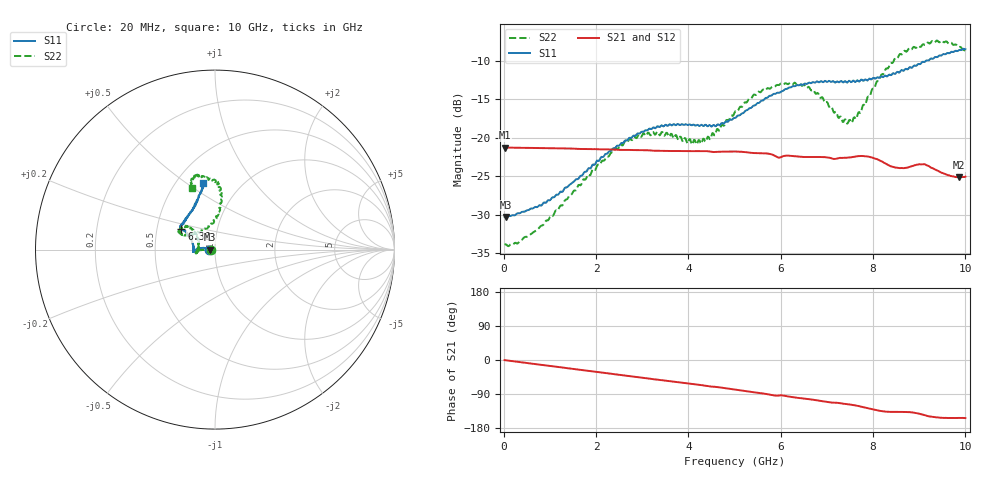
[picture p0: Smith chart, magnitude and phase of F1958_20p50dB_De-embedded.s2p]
! Integrated Device Technology
! Corporate Headquarters
! 6024 Silver Creek Valley Road
! San Jose, CA 95138  USA
! Phone:  1-408-284-8200
! Toll Free:  1-800-223-1366
! Webpage:  http://www.idt.com/
! Timing and RF Division
! 515 Groton Road, Suite 102
! Westford, MA 01886-6024
! Device:  F1958
! Description: 7-bit 0.25 dB Digital Step Attenuator
! Frequency:  0.001 -  6.000 GHz
! Package:  4x4 mm Thin QFN Plastic Package: 24 pin
! Ports:  2 RF, 12 DC
!  Pin  1  = D0
!  Pin  2  = VDD
!  Pin  3  = VMODE
!  Pin  4  = GND
!  Pin  5  = RF1  =  Port 1
!  Pin  6  = GND
!  Pin  7  = GND
!  Pin  8  = GND
!  Pin  9  = GND
!  Pin 10  = GND
!  Pin 11  = GND
!  Pin 12  = GND
!  Pin 13  = GND
!  Pin 14  = RF2  =  Port 2
!  Pin 15  = GND
!  Pin 16  = LE
!  Pin 17  = CLK
!  Pin 18  = DATA
!  Pin 19  = D6
!  Pin 20  = D5
!  Pin 21  = D4
!  Pin 22  = D3
!  Pin 23  = D2
!  Pin 24  = D1
! State:  82
! Atten State:  20.50 dB
! Voltage:  +3.30 Volts
! Current:  0.258 mA
! Data:  The device was measured on a F1958 evaluation board which has
!  individual transmission lines to the RF pins.  Data was collected
!  using a calibrated network analyzer.  The evaluation board was
!  de-embedded using Automatic Fixture Removal (AFR).
!  The reference plane is the edge of the package pin.
! Misc:
!  Action Tracker AT0419
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# GHz S dB R 50
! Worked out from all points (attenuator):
!   500 points, 20 MHz to 10 GHz, reference 50 ohm
!   highest |S21| = -21.27 dB at 20 MHz (marker M1); lowest = -25.1 dB at 9.86 GHz (marker M2)
!   lowest |S11| = -30.3 dB at 40 MHz (marker M3), VSWR 1.06, Z = 47 - j0.042 ohm
!   |S11| at or under -10 dB: start of sweep to 9.144 GHz
!   |S22| runs from -34.1 to -7.3 dB; largest |S21 - S12| = 0.00033
!   S11 on the Smith chart (normalised r, x): 20 MHz: 0.94, -0.00; 6.36 GHz: 0.67, +0.16; 10 GHz: 0.68, +0.58
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0.02  -30.27 -178.9  -21.27 -0.4  -21.27 -0.4  -33.91 -178.0
0.04  -30.30 -179.2  -21.27 -0.7  -21.27 -0.7  -33.85 -177.0
0.32  -29.82 175.3  -21.31 -5.1  -21.30 -5.1  -33.64 178.7
0.72  -29.03 172.9  -21.33 -11.4  -21.33 -11.4  -31.97 180.0
1.7  -24.90 171.4  -21.45 -26.5  -21.45 -26.5  -25.75 179.3
2.6  -20.60 177.3  -21.58 -40.4  -21.56 -40.4  -20.76 -176.4
3.36  -18.59 -175.3  -21.70 -52.3  -21.70 -52.4  -19.52 -168.5
4.24  -18.48 -178.7  -21.74 -65.7  -21.75 -65.7  -20.32 169.3
4.52  -18.48 174.4  -21.86 -70.2  -21.87 -70.3  -19.39 153.9
5.02  -17.41 161.1  -21.79 -78.0  -21.81 -78.0  -16.53 139.4
5.58  -15.17 150.8  -22.01 -87.5  -22.03 -87.6  -13.99 139.6
6.36  -13.15 148.2  -22.44 -99.8  -22.46 -99.7  -13.15 153.1
6.68  -12.81 146.7  -22.49 -104.5  -22.51 -104.4  -13.81 154.3
7.3  -12.61 140.9  -22.62 -114.3  -22.62 -114.1  -17.24 134.0
7.5  -12.64 138.3  -22.57 -117.5  -22.56 -117.4  -17.67 115.5
7.68  -12.60 135.4  -22.39 -121.4  -22.39 -121.3  -16.71 98.0
8.34  -11.81 119.2  -23.58 -136.8  -23.58 -136.9  -10.81 82.6
8.68  -11.18 112.5  -23.94 -137.3  -23.95 -137.1  -8.68 87.1
9.06  -10.16 106.9  -23.46 -143.7  -23.47 -143.7  -7.97 95.2
9.26  -9.69 104.8  -23.90 -149.6  -23.89 -149.8  -7.54 100.1
9.86  -8.61 99.9  -25.14 -152.9  -25.18 -152.9  -8.19 109.2
10  -8.48 99.9  -25.05 -153.2  -25.10 -153.2  -8.70 110.1
